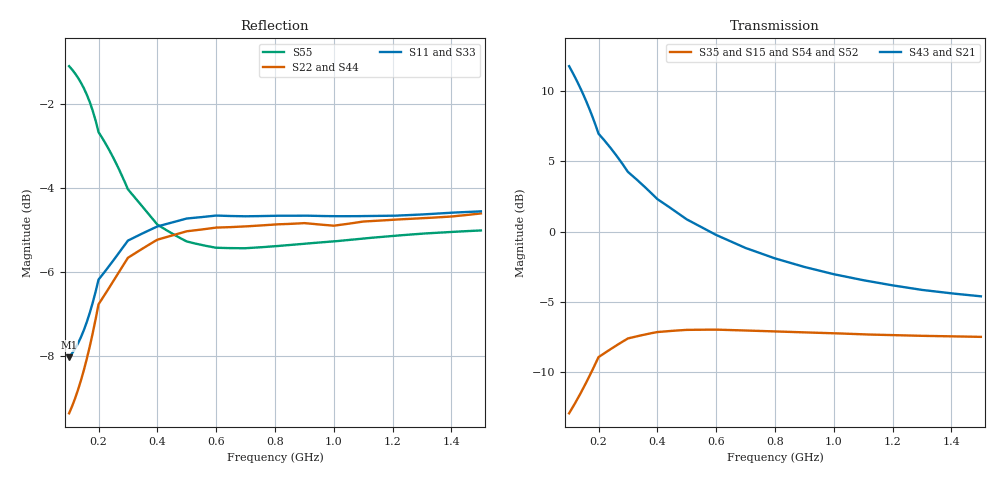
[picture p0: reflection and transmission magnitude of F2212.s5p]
! Date: Tue Aug 08 14:34:49 1995
!  POLYFET RF DEVICES
!  F2212
!  S PARAMETERS
!  VDS=12.5V, IDQ=800mA
!AWR Design Environment (2053) Thu Feb 05 14:07:31 2004
!freq-unit  param-type  data-format  keyword  impedance-ohms
# MHz  S  MA  R  50
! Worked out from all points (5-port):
!   141 points, 100 MHz to 1.5 GHz, reference 50 ohm
!   strongest paths, dB at 100 MHz, 450 MHz, 800 MHz, 1.15 GHz, 1.5 GHz:
!     S43: 11.8, 1.6, -1.9, -3.6, -4.6
!     S21: 11.8, 1.6, -1.9, -3.6, -4.6
!     S35: -12.9, -7.1, -7.1, -7.3, -7.5
!     S15: -12.9, -7.1, -7.1, -7.3, -7.5
!     S54: -13.0, -7.2, -7.2, -7.4, -7.6
!     S52: -13.0, -7.2, -7.2, -7.4, -7.6
!   lowest |S11| = -8.0 dB at 100 MHz (marker M1), VSWR 2.32, Z = 33.3 - j31.1 ohm
!   |S11| at or under -10 dB: nowhere
